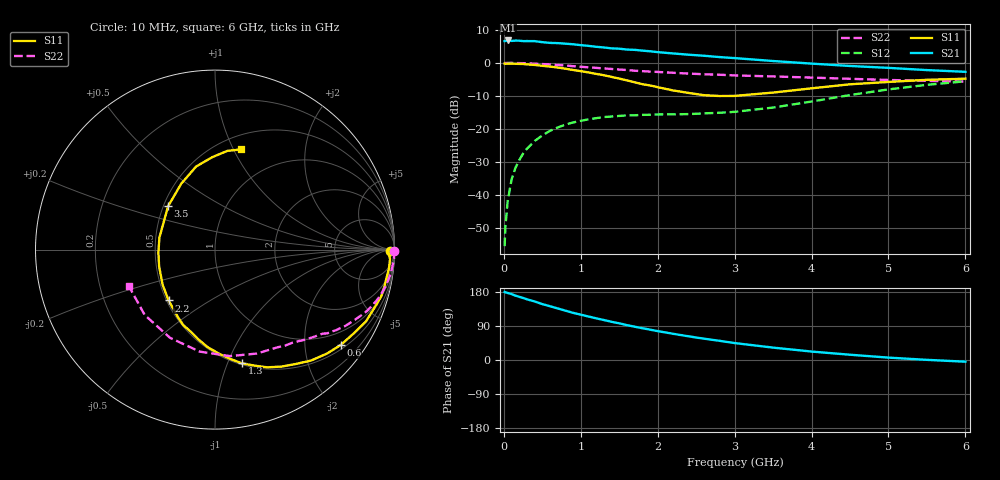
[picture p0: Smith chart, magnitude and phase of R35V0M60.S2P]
! SIEMENS Small Signal Semiconductors
! BFR181
! Si NPN RF Bipolar Junction Transistor in SOT23
! VCE = 5 V  IC = 0.6 mA
! Common Emitter S-Parameters:  May  1996
# GHz  S  MA  R  50
!  f  S11  S21  S12  S22
! GHz  MAG  ANG  MAG  ANG  MAG  ANG  MAG  ANG
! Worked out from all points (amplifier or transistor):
!   36 points, 10 MHz to 6 GHz, reference 50 ohm
!   highest |S21| = 6.8 dB at 50 MHz (marker M1)
!   |S21| within 3 dB of that: start of sweep to 1.769 GHz
!   unconditionally stable (mu >= 1): 2.292 GHz to 3.882 GHz
!   at 250 MHz: K = 0.13, MSG = 17.0 dB, |S12| = -27.4 dB
!   at 1.4 GHz: K = 0.64, MSG = 10.3 dB, |S12| = -16.2 dB
!   at 6 GHz: K = 0.91, MSG = 1.4 dB, |S12| = -5.6 dB
!   S11 on the Smith chart (normalised r, x): 10 MHz: 70, -31; 600 MHz: 0.61, -2.86; 1.3 GHz: 0.51, -1.13; 2.2 GHz: 0.51, -0.34; 3.5 GHz: 0.53, +0.29; 6 GHz: 0.64, +1.07
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0.01  0.9763 -0.6  2.133 179.6  0.0017 90.5  0.9988 -0.3
0.02  0.9672 -1.1  2.137 178.6  0.0033 90.0  0.9939 -0.6
0.05  0.9767 -3.1  2.182 176.9  0.0082 87.8  0.9974 -1.5
0.1  0.9749 -6.3  2.146 174.0  0.0172 85.8  0.9988 -2.9
0.15  0.9685 -9.5  2.171 169.8  0.0258 83.0  0.9946 -4.6
0.25  0.9621 -15.7  2.134 163.7  0.0425 78.6  0.9885 -7.5
0.4  0.9314 -25.5  2.132 154.5  0.0659 73.0  0.9739 -11.8
0.5  0.9027 -31.2  2.056 147.5  0.0801 69.0  0.96 -14.6
0.6  0.8794 -37.2  2.005 141.9  0.0941 65.0  0.9468 -17.1
0.7  0.8511 -42.9  1.989 136.1  0.1056 61.7  0.9297 -19.6
0.9  0.7813 -54.6  1.911 124.4  0.1257 54.9  0.8924 -24.3
1.1  0.7175 -66.1  1.809 114.8  0.1402 49.3  0.8568 -28.4
1.3  0.651 -76.7  1.71 105.5  0.1516 44.7  0.8245 -32.0
1.7  0.5092 -100.4  1.574 87.9  0.1614 39.1  0.761 -38.0
2  0.4296 -118.7  1.453 76.2  0.1663 37.2  0.7298 -42.1
2.2  0.3832 -132.4  1.389 69.2  0.1668 37.1  0.7088 -45.1
2.6  0.3253 -163.1  1.282 56.3  0.1726 39.6  0.6733 -50.6
3  0.3169 167.9  1.181 44.7  0.182 43.7  0.6465 -57.3
3.5  0.3559 137.3  1.067 32.7  0.2114 48.9  0.6242 -68.1
4.5  0.4747 102.8  0.898 13.9  0.3264 49.6  0.5747 -98.5
5.5  0.5547 82.8  0.778 0.4  0.4657 37.2  0.5349 -137.1
6  0.577 75.3  0.733 -4.5  0.527 28.8  0.5215 -157.3
